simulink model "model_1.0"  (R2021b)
settings: Solver=VariableStepAuto  StartTime=0.0  StopTime=20  RelTol=1e-3
libraries: fl_lib x20, nesl_utility x8, simulink x1, sdl_lib x1

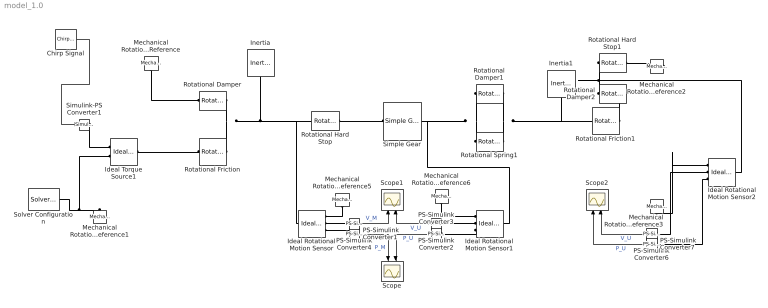
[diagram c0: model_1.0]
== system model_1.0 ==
  Chirp Signal : simulink/Sources/Chirp Signal  f1=0.1  T=10  f2=1
  Ideal Rotational Motion Sensor : fl_lib/Mechanical/Mechanical Sensors/Ideal Rotational Motion Sensor  wrap_angle=simscape.enum.onoff.off  offset=0 rad
  Ideal Rotational Motion Sensor1 : fl_lib/Mechanical/Mechanical Sensors/Ideal Rotational Motion Sensor  wrap_angle=simscape.enum.onoff.off  offset=0 rad
  Ideal Rotational Motion Sensor2 : fl_lib/Mechanical/Mechanical Sensors/Ideal Rotational Motion Sensor  wrap_angle=simscape.enum.onoff.off  offset=0 rad
  Ideal Torque Source1 : fl_lib/Mechanical/Mechanical Sources/Ideal Torque Source
  Inertia : fl_lib/Mechanical/Rotational Elements/Inertia  inertia=0.085 kg*m^2  num_ports=foundation.enum.numPorts2.one  w_specify=off  w_priority=High  w=0 rad/s  w_nominal_specify=off  w_nominal_unit=rad/s  w_nominal_value=1  t_specify=off  t_priority=None  t=0 N*m  t_nominal_specify=off  t_nominal_unit=N*m  t_nominal_value=1
  Inertia1 : fl_lib/Mechanical/Rotational Elements/Inertia  inertia=50 kg*m^2  num_ports=foundation.enum.numPorts2.one  w_specify=off  w_priority=High  w=0 rad/s  w_nominal_specify=off  w_nominal_unit=rad/s  w_nominal_value=1  t_specify=off  t_priority=None  t=0 N*m  t_nominal_specify=off  t_nominal_unit=N*m  t_nominal_value=1
  Mechanical Rotational Reference{,1..3,5..6} (6 alike) : fl_lib/Mechanical/Rotational Elements/Mechanical Rotational Reference
  PS-Simulink Converter{1..4,6..7} (6 alike) : nesl_utility/PS-Simulink Converter  PhysicalDomain=network_engine_domain  SubClassName=ps_output  LeftPortType=input  RightPortType=output  PseudoPeriodic=off  Frequencies=[]  Unit=inherit  AffineConversion=off
  Rotational Damper : fl_lib/Mechanical/Rotational Elements/Rotational Damper  D=0.03 N*m/(rad/s)  w_specify=off  w_priority=None  w=0 rad/s  w_nominal_specify=off  w_nominal_unit=rad/s  w_nominal_value=1  t_specify=off  t_priority=None  t=0 N*m  t_nominal_specify=off  t_nominal_unit=N*m  t_nominal_value=1
  Rotational Damper1 : fl_lib/Mechanical/Rotational Elements/Rotational Damper  D=50 N*m/(rad/s)  w_specify=off  w_priority=None  w=0 rad/s  w_nominal_specify=off  w_nominal_unit=rad/s  w_nominal_value=1  t_specify=off  t_priority=None  t=0 N*m  t_nominal_specify=off  t_nominal_unit=N*m  t_nominal_value=1
  Rotational Damper2 : fl_lib/Mechanical/Rotational Elements/Rotational Damper  D=100 N*m/(rad/s)  w_specify=off  w_priority=None  w=0 rad/s  w_nominal_specify=off  w_nominal_unit=rad/s  w_nominal_value=1  t_specify=off  t_priority=None  t=0 N*m  t_nominal_specify=off  t_nominal_unit=N*m  t_nominal_value=1
  Rotational Friction : fl_lib/Mechanical/Rotational Elements/Rotational Friction  brkwy_trq=5 N*m  brkwy_vel=0.1 rad/s  Col_trq=5 N*m  visc_coef=0 N*m/(rad/s)  w_specify=off  w_priority=None  w=0 rad/s  w_nominal_specify=off  w_nominal_unit=rad/s  w_nominal_value=1  t_specify=off  t_priority=None  t=0 N*m  t_nominal_specify=off  t_nominal_unit=N*m  t_nominal_value=1
  Rotational Friction1 : fl_lib/Mechanical/Rotational Elements/Rotational Friction  brkwy_trq=500 N*m  brkwy_vel=0.1 rad/s  Col_trq=500 N*m  visc_coef=0 N*m/(rad/s)  w_specify=off  w_priority=None  w=0 rad/s  w_nominal_specify=off  w_nominal_unit=rad/s  w_nominal_value=1  t_specify=off  t_priority=None  t=0 N*m  t_nominal_specify=off  t_nominal_unit=N*m  t_nominal_value=1
  Rotational Hard Stop : fl_lib/Mechanical/Rotational Elements/Rotational Hard Stop  upper_bnd=1 deg  lower_bnd=-1 deg  stiff_up=1e6 N*m/rad  stiff_low=1e6 N*m/rad  D_up=0.01 N*m/(rad/s)  D_low=0.01 N*m/(rad/s)  model=simscape.enum.hardstop.smooth  transition=0.001 rad  w_specify=off  w_priority=None  w=0 rad/s  w_nominal_specify=off  w_nominal_unit=rad/s  w_nominal_value=1  t_specify=off  t_priority=None  t=0 N*m  t_nominal_specify=off  t_nominal_unit=N*m  t_nominal_value=1  phi_specify=off  phi_priority=High  phi=0 rad  phi_nominal_specify=off  phi_nominal_unit=rad  phi_nominal_value=1
  Rotational Hard Stop1 : fl_lib/Mechanical/Rotational Elements/Rotational Hard Stop  upper_bnd=45 deg  lower_bnd=-45 deg  stiff_up=1e6 N*m/rad  stiff_low=1e6 N*m/rad  D_up=0.01 N*m/(rad/s)  D_low=0.01 N*m/(rad/s)  model=simscape.enum.hardstop.smooth  transition=0.001 rad  w_specify=off  w_priority=None  w=0 rad/s  w_nominal_specify=off  w_nominal_unit=rad/s  w_nominal_value=1  t_specify=off  t_priority=None  t=0 N*m  t_nominal_specify=off  t_nominal_unit=N*m  t_nominal_value=1  phi_specify=off  phi_priority=High  phi=0 rad  phi_nominal_specify=off  phi_nominal_unit=rad  phi_nominal_value=1
  Rotational Spring1 : fl_lib/Mechanical/Rotational Elements/Rotational Spring  spr_rate=50 N*m/rad  w_specify=off  w_priority=None  w=0 rad/s  w_nominal_specify=off  w_nominal_unit=rad/s  w_nominal_value=1  t_specify=off  t_priority=None  t=0 N*m  t_nominal_specify=off  t_nominal_unit=N*m  t_nominal_value=1  phi_specify=off  phi_priority=High  phi=0 rad  phi_nominal_specify=off  phi_nominal_unit=rad  phi_nominal_value=1
  Scope : Scope  NumInputPorts=2
  Scope1 : Scope  NumInputPorts=2
  Scope2 : Scope  NumInputPorts=2
  Simple Gear : sdl_lib/Gears/Simple Gear  ratio=100  rotation_direction=sdl.enum.shaftOutputDirection.same  friction_model=sdl.enum.gear_efficiencies_load.off  T_noload=0.1 N*m  T_nom=5 N*m  efficiency_nom=0.8  efficiency=0.8  temperature_TLU=[280, 300, 320] K  load_TLU=[1, 5, 10] N*m  efficiency_TLU=[.95, .9, .85]  efficiency_TLU2=[.85, .8, .75; .95, .9, .85; .85, .8, .7]  w_thr=0.01 rad/s  pwr_thr=0.001 W  backlash_model=sdl.enum.backlashModel.Off  backlash_distance=1e-3 mm  x0=0 mm  r_base=0.1 m  hardstop_model=simscape.enum.hardstop.smooth  transition=1e-4 mm  backlash_stiffness=1e7 N/m  backlash_damping=1e6 N/(m/s)  e=0  v_tol=0.001 m/s  mu_visc=[0, 0] N*m/(rad/s)  enable_faults=simscape.enum.onoff.off  efficiency_fault=0.05  external_fault=simscape.enum.onoff.off  temporal_fault=simscape.enum.onoff.off  fault_time=5 s  fault_angles=pi / 12 rad  report_fault=simscape.enum.assert.action.none  thermal_mass=50 J/K  temperature_specify=off  temperature_priority=High  temperature=300 K  temperature_nominal_specify=off  temperature_nominal_unit=K  temperature_nominal_value=1
  Simulink-PS Converter1 : nesl_utility/Simulink-PS Converter  PhysicalDomain=network_engine_domain  SubClassName=ps_input  LeftPortType=input  RightPortType=output  PseudoPeriodic=off  Frequencies=[]  NoiseDistribution=none  NoiseParameters=[]  Unit=1  AffineConversion=off  FilteringAndDerivatives=provide  SimscapeFilterOrder=1  InputFilterTimeConstant=0.001  UdotUserProvided=0
  Solver Configuration : nesl_utility/Solver Configuration  PhysicalDomain=network_engine_domain  SubClassName=solver  LeftPortType=input  RightPortType=generic  Tones=[]  Harmonics=[]  SimulateNoise=off  Profile=off  UseLocalSampling=off  EnableSwitchedLinearOptims=on  FrequencyDomain=off  UseCCode=off  RelTol=0.001  AbsTol=1e-06  MinStep=1e-09  ToWorkspace=off  RevertToSquareIcSolve=off  NumHomotopyIterations=100  PhasorMode=off  PhasorModeNumHarmonics=1  DoDC=off  ResidualTolerance=1e-09  UseLocalSolver=off  LocalSolverChoice=NE_BACKWARD_EULER_ADVANCER  LocalSolverSampleTime=0.001  DoFixedCost=off  MaxNonlinIter=3  MaxModeIter=2  ComputeImpulses=off  ImpulseIterations=2  LinearAlgebra=auto  EquationFormulation=NE_TIME_EF  DelaysMemoryBudget=1024  AutomaticFiltering=on  FilteringTimeConstant=0.001  PartitionStorageMethod=AS_NEEDED  PartitionMemoryBudget=1024  PartitionMethod=ROBUST
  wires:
  PS-Simulink Converter2/1 -> Scope1/2  "V_U"
  PS-Simulink Converter4/1 -> Scope1/1  "V_M"
  PS-Simulink Converter3/1 -> Scope/2  "P_U"
  PS-Simulink Converter1/1 -> Scope/1  "P_M"
  PS-Simulink Converter6/1 -> Scope2/2  "V_U"
  PS-Simulink Converter7/1 -> Scope2/1  "P_U"
  Chirp Signal/1 -> Simulink-PS Converter1/1
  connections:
  Mechanical Rotational Reference/LConn1 -- Rotational Damper/LConn1
  Ideal Torque Source1/LConn1 -- Rotational Friction/LConn1
  Rotational Friction/RConn1 -- Ideal Rotational Motion Sensor/LConn1 -- Rotational Hard Stop/LConn1 -- Inertia/LConn1 -- Rotational Damper/RConn1
  Mechanical Rotational Reference1/LConn1 -- Solver Configuration/RConn1 -- Ideal Torque Source1/RConn2
  Rotational Hard Stop/RConn1 -- Simple Gear/LConn1
  Rotational Damper1/LConn1 -- Ideal Rotational Motion Sensor1/LConn1 -- Simple Gear/RConn1 -- Rotational Spring1/LConn1
  Rotational Damper1/RConn1 -- Inertia1/LConn1 -- Rotational Friction1/LConn1 -- Rotational Spring1/RConn1
  Rotational Damper2/RConn1 -- Rotational Friction1/RConn1
  Ideal Rotational Motion Sensor1/RConn3 -- PS-Simulink Converter3/LConn1
  PS-Simulink Converter2/LConn1 -- Ideal Rotational Motion Sensor1/RConn2
  Mechanical Rotational Reference5/LConn1 -- Ideal Rotational Motion Sensor/RConn1
  Mechanical Rotational Reference6/LConn1 -- Ideal Rotational Motion Sensor1/RConn1
  PS-Simulink Converter1/LConn1 -- Ideal Rotational Motion Sensor/RConn3
  PS-Simulink Converter4/LConn1 -- Ideal Rotational Motion Sensor/RConn2
  Rotational Hard Stop1/LConn1 -- Ideal Rotational Motion Sensor2/LConn1 -- Rotational Damper2/LConn1
  Mechanical Rotational Reference2/LConn1 -- Rotational Hard Stop1/RConn1
  Mechanical Rotational Reference3/LConn1 -- Ideal Rotational Motion Sensor2/RConn1
  Ideal Rotational Motion Sensor2/RConn3 -- PS-Simulink Converter7/LConn1
  PS-Simulink Converter6/LConn1 -- Ideal Rotational Motion Sensor2/RConn2
  Simulink-PS Converter1/RConn1 -- Ideal Torque Source1/RConn1
